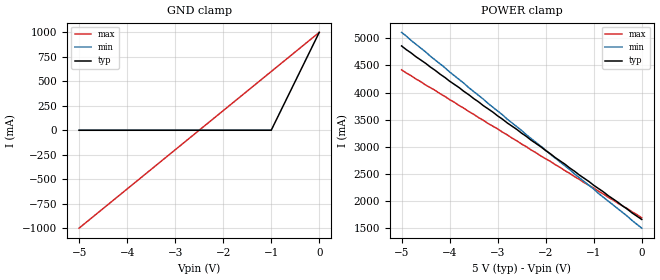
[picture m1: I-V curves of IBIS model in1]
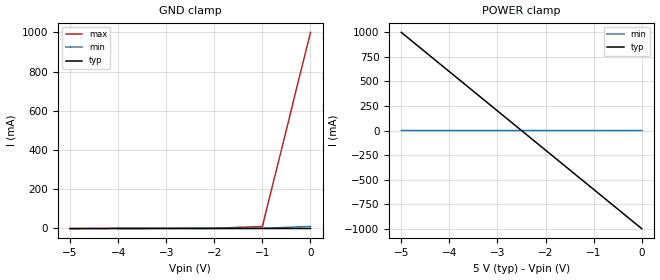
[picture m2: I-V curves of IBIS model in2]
|   Parser fails to detect and report clamp I-V tables where current always
|   flows.
[IBIS Ver]   2.1
[File Name]   bug56.ibs
[File Rev]   0.1
[Component]   TEST
[Manufacturer]   Test File
[Package]
| variable   typ   min   max
R_pkg   0.0m   NA   NA
L_pkg   0.0nH   NA   NA
C_pkg   0.0pF   NA   NA
[Pin]   signal_name   model_name
1   One_Pin   in1
2   Two_Pin   in2
| Models and submodels in the file (2): in1 (Input), in2 (Input)
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[Model]   in1
Model_type   Input
Vinl =   0.80V
Vinh =   2.00V
C_comp   2.00pF   1.00pF   3.00pF
[Temperature Range]   50.00   100.00   0.000
[Voltage Range]   5.00V   4.50V   5.50V
| .. all these curves should generate warnings
[POWER_clamp]
| voltage   I(typ)   I(min)   I(max)
-5V       4.86A      5.11A      4.42A
-2.4V     3.19A      3.22A      3A
-1.3V     2.48A      2.43A      2.4A
0V        1.66A      1.5A       1.69A
[GND_clamp]
| ... typ crv is within zero threshold
| ... min crv is invalid so don't warn even if the crv never touches zero
| ... max crv has a sign change so assume it crosses zero
| voltage   I(typ)   I(min)   I(max)
-5V       10nA       10uA       -1A
-4V       100nA      10uA       NA
-2V       1uA        100uA      NA
-1V       10uA       1mA        NA
0V        1A         NA         1A
[Model]   in2
Model_type   Input
Vinl =   0.80V
Vinh =   2.00V
C_comp   2.00pF   1.00pF   3.00pF
[Temperature Range]   50.00   100.00   0.000
[Voltage Range]   5.00V   4.50V   5.50V
[POWER_clamp]
| ... typ crv has a sign change so assume it crosses zero
| ... min crv is within zero threshold
| ... max crv has no values so don't check for zero threshold
| voltage   I(typ)   I(min)   I(max)
-5V       1A         10uA       NA
-100mV    NA         1uA        NA
0V        -1A        0A         NA
[GND_clamp]
| ... typ crv is within negative threshold
| ... min crv is invalid so don't warn even if the crv never touches zero
| ... max crv should generate a warning
| voltage   I(typ)   I(min)   I(max)
-5V       -1mA       NA         9uA
-4V       -100uA     10uA       100uA
-2V       -10uA      100uA      1mA
-1V       -1uA       1mA        10mA
0V        -1uA       10mA       1A
